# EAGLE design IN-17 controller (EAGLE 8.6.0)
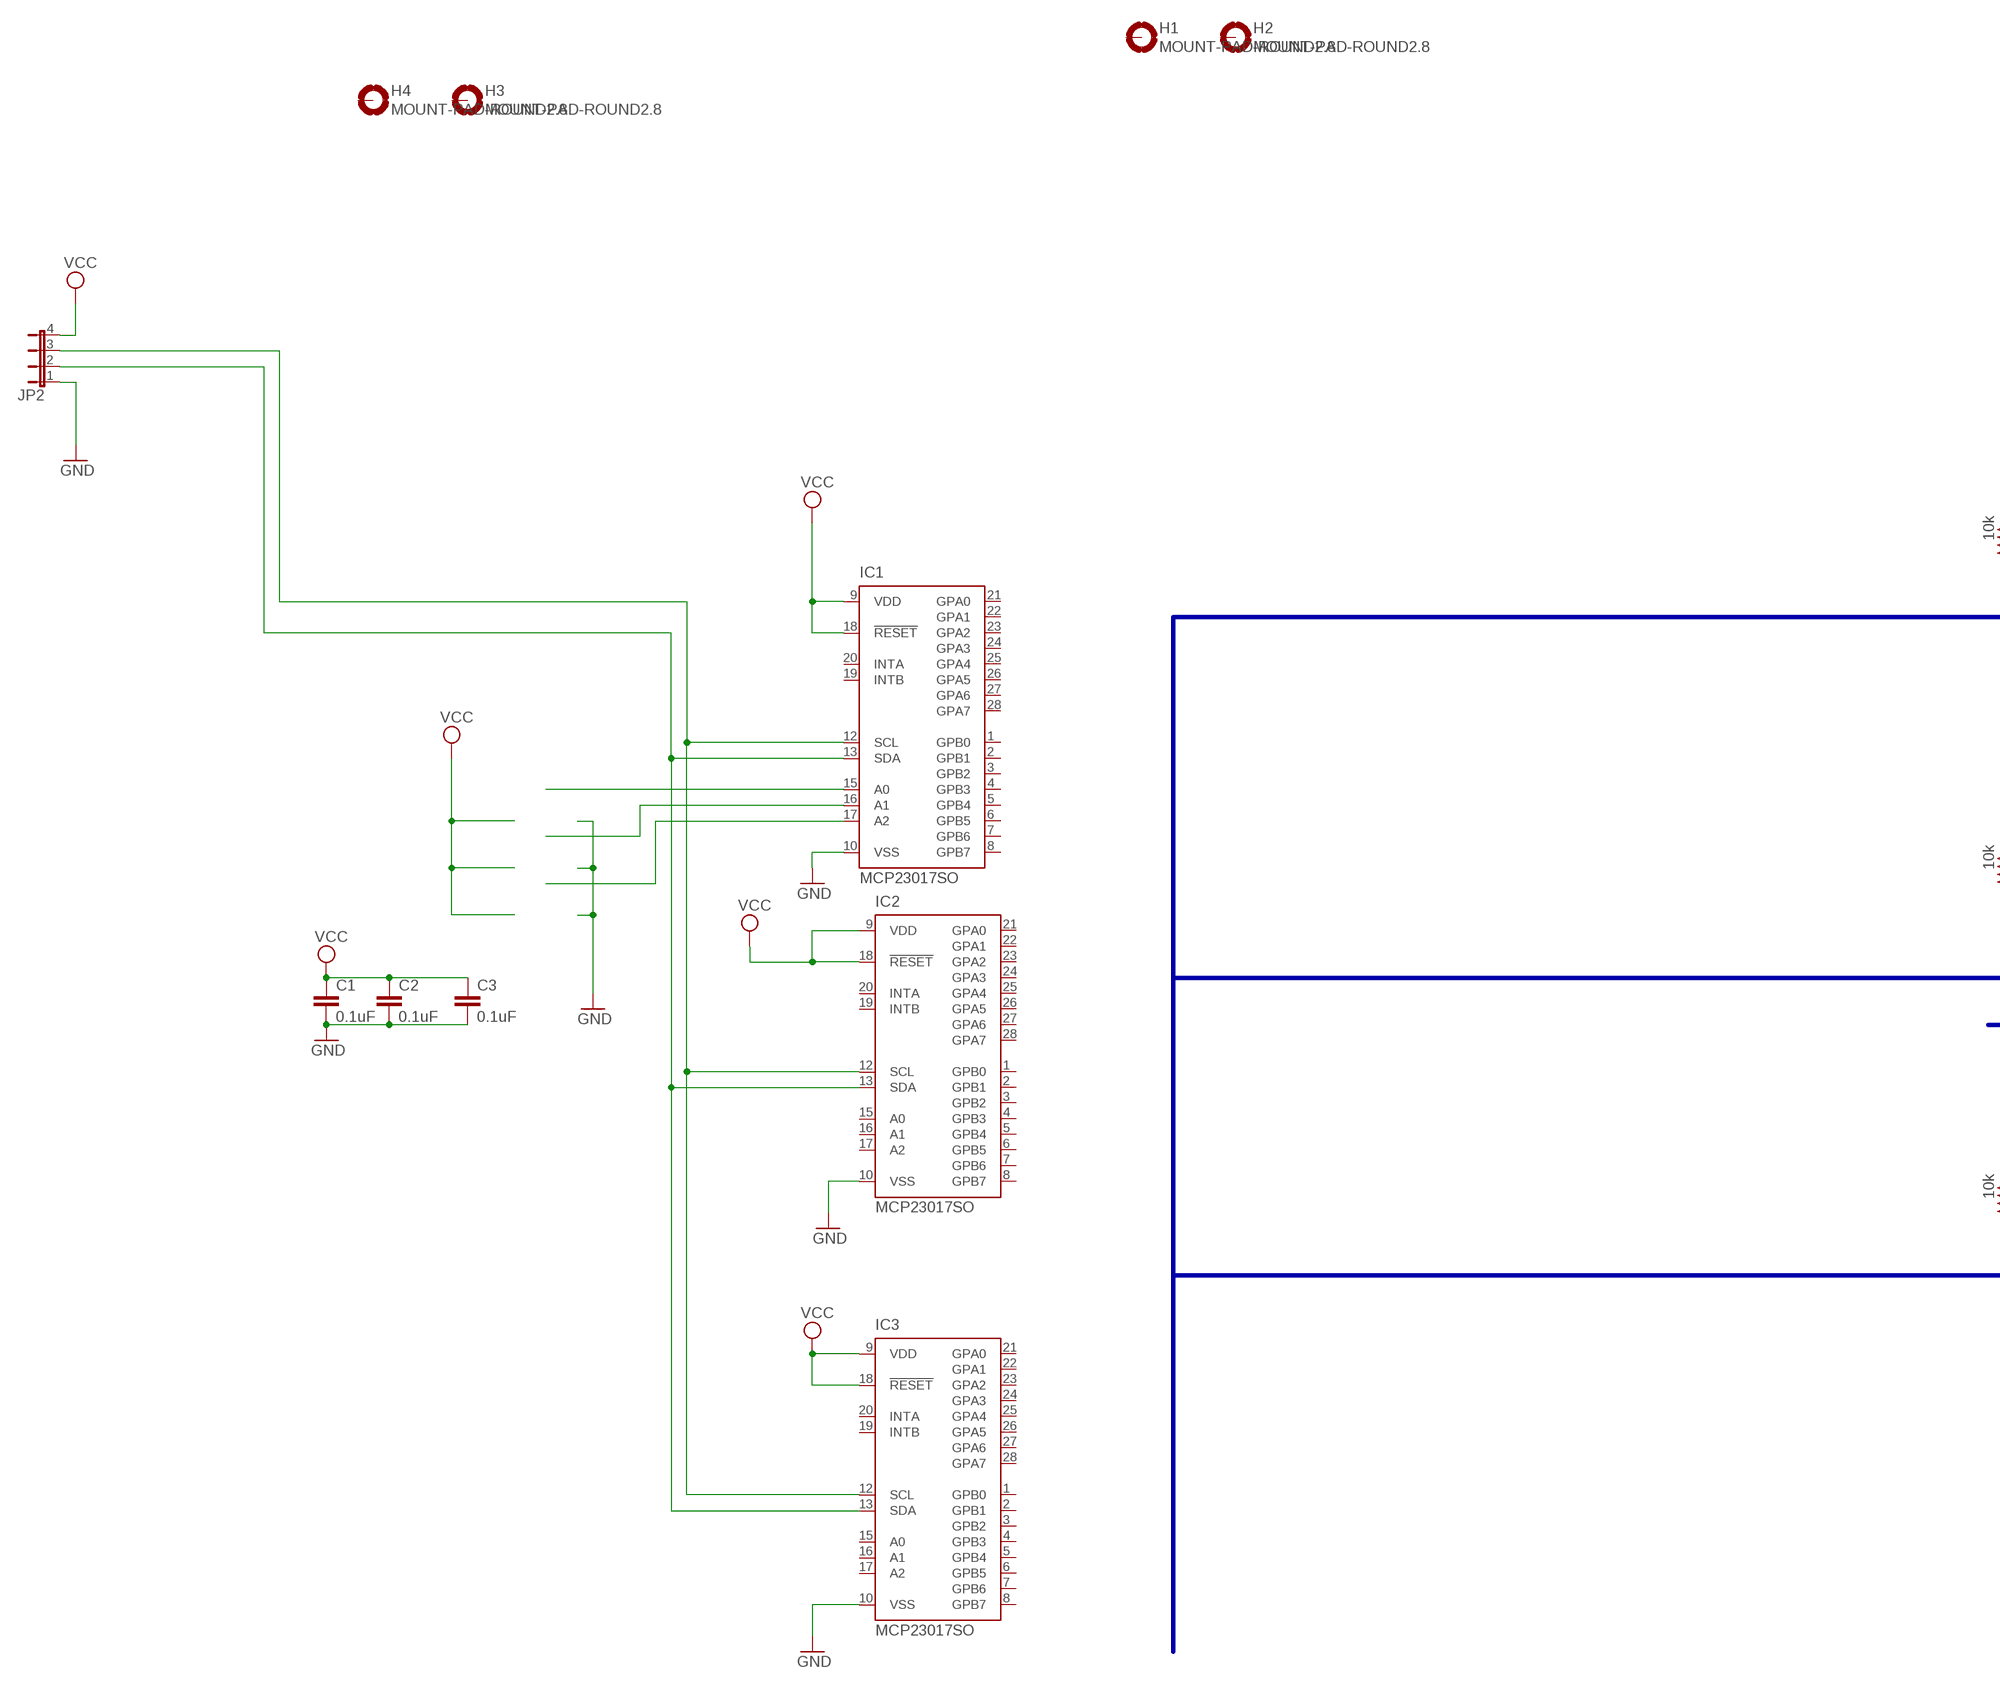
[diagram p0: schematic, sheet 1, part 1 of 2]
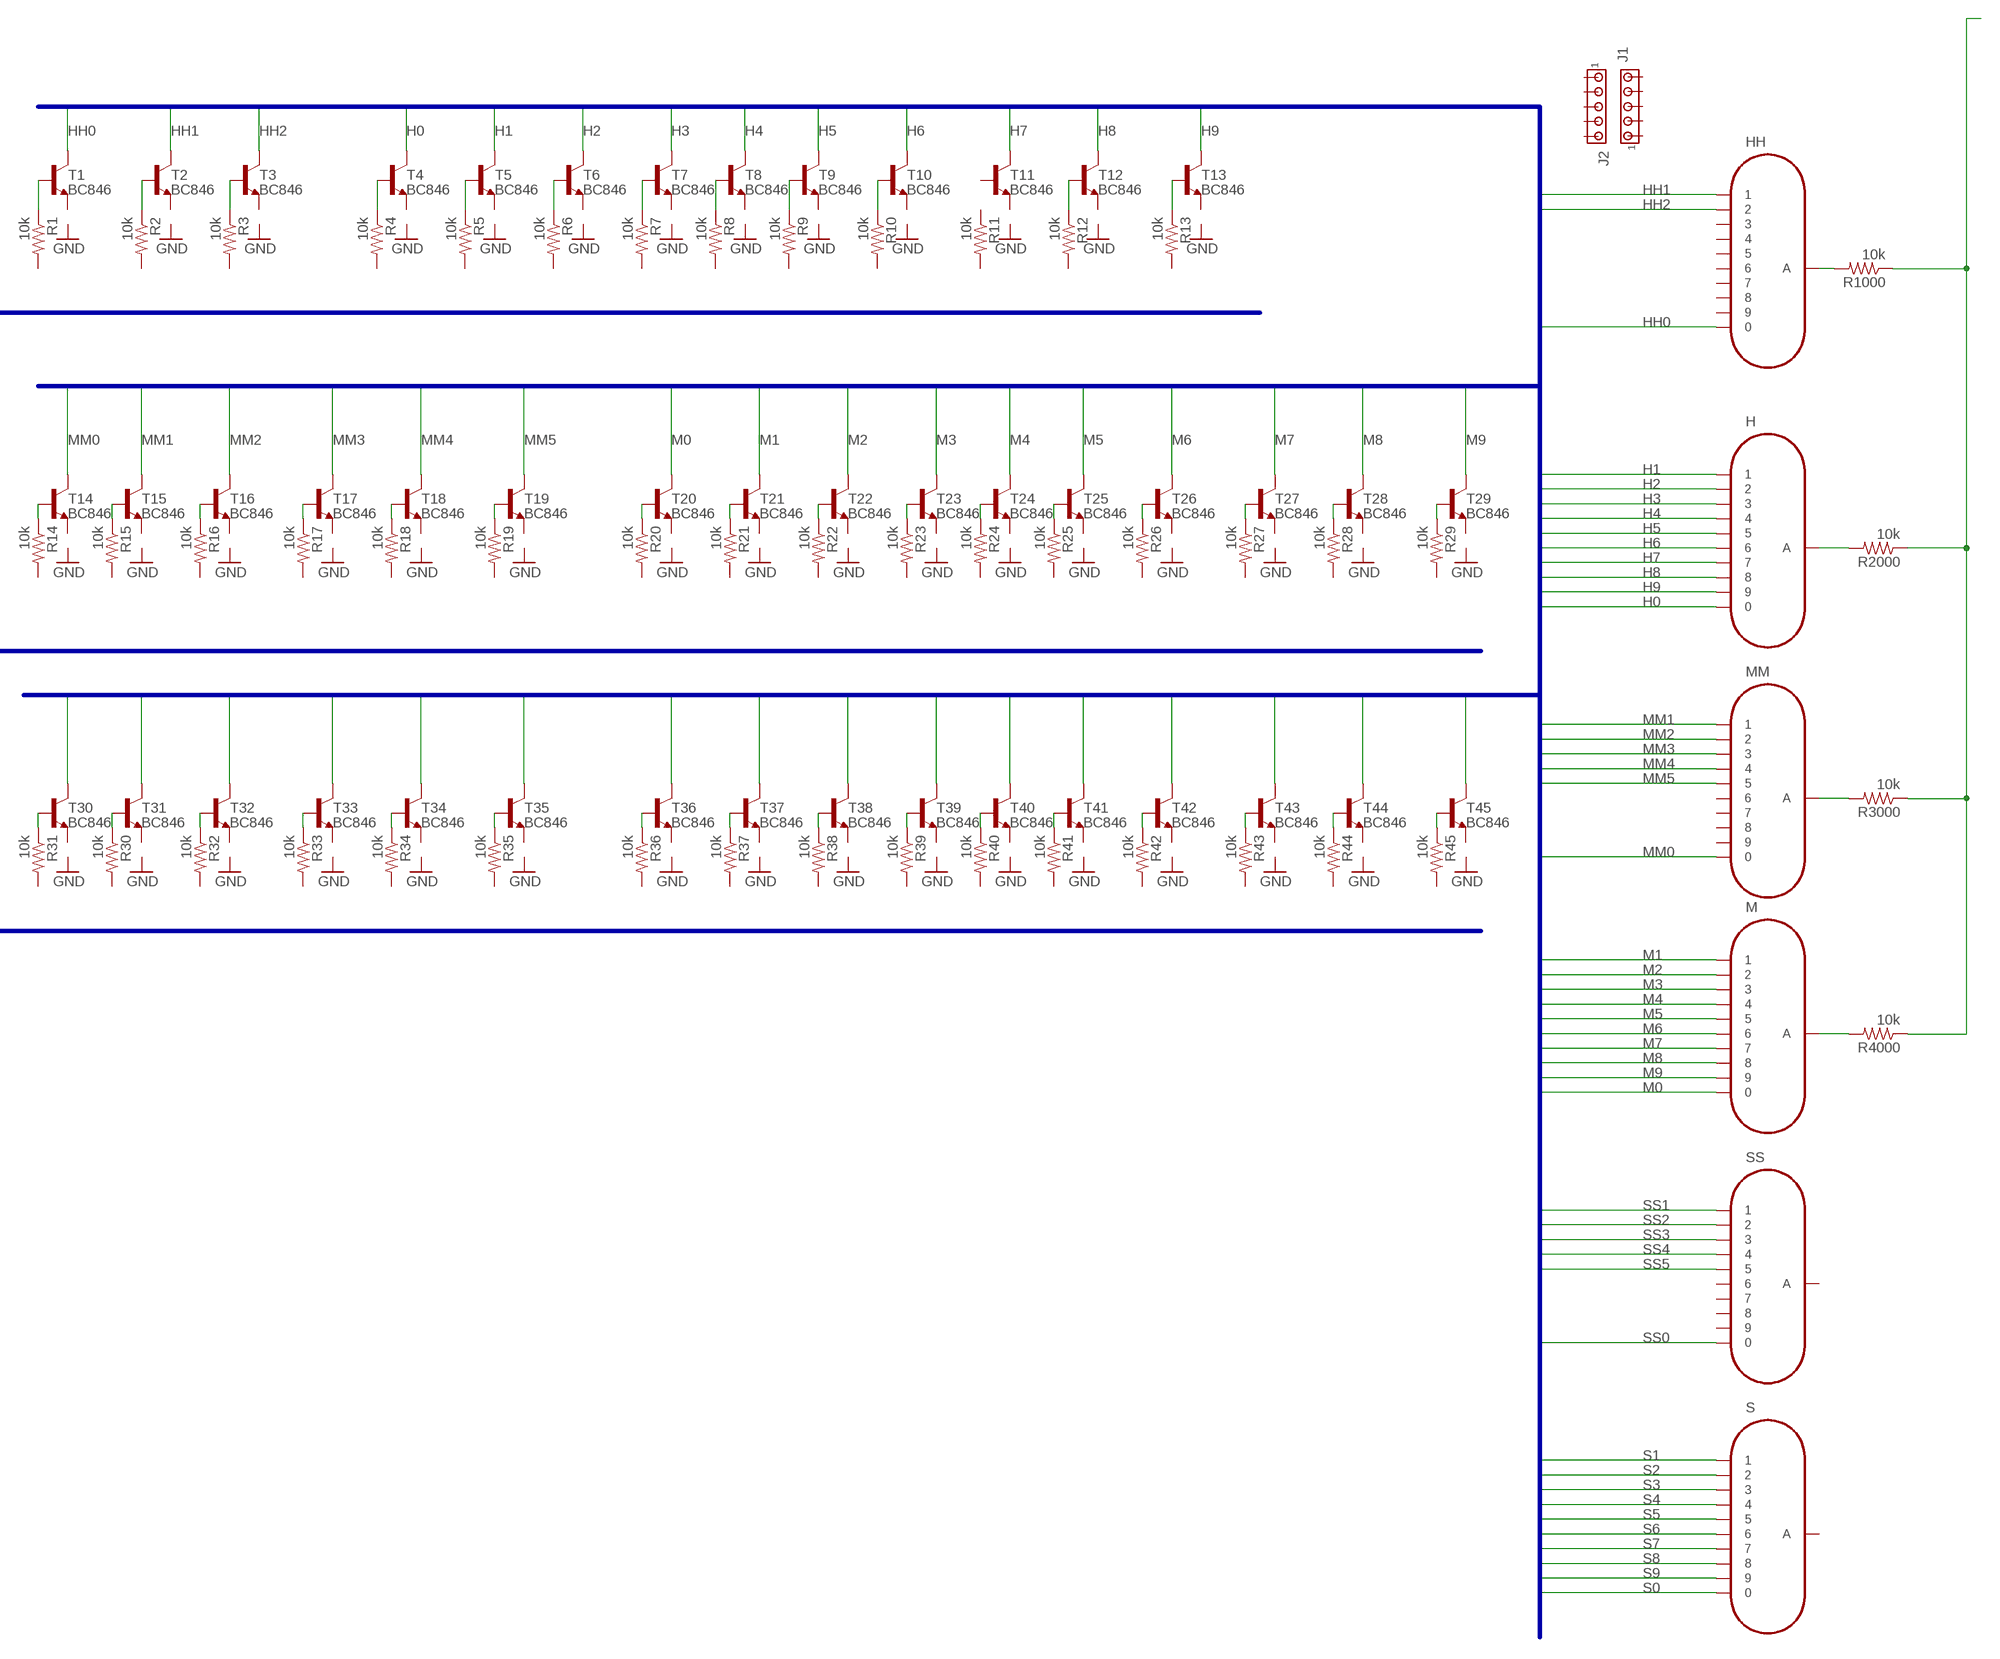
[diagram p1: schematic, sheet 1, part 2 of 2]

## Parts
C1  0.1uF  C-EUC1206  [C1206]
C2  0.1uF  C-EUC1206  [C1206]
C3  0.1uF  C-EUC1206  [C1206]
H  IN-17  [IN-17]
H1  MOUNT-PAD-ROUND2.8  [2,8-PAD]
H2  MOUNT-PAD-ROUND2.8  [2,8-PAD]
H3  MOUNT-PAD-ROUND2.8  [2,8-PAD]
H4  MOUNT-PAD-ROUND2.8  [2,8-PAD]
HH  IN-17  [IN-17]
IC1  MCP23017SO  [SO28W]
IC2  MCP23017SO  [SO28W]
IC3  MCP23017SO  [SO28W]
J1  MTA05-100  [10X05MTA]
J2  MTA05-100  [10X05MTA]
JP2  JP4E  [JP4]
M  IN-17  [IN-17]
MM  IN-17  [IN-17]
R1  10k  R-US_M0805  [M0805]
R2  10k  R-US_M0805  [M0805]
R3  10k  R-US_M0805  [M0805]
R4  10k  R-US_M0805  [M0805]
R5  10k  R-US_M0805  [M0805]
R6  10k  R-US_M0805  [M0805]
R7  10k  R-US_M0805  [M0805]
R8  10k  R-US_M0805  [M0805]
R9  10k  R-US_M0805  [M0805]
R10  10k  R-US_M0805  [M0805]
R11  10k  R-US_M0805  [M0805]
R12  10k  R-US_M0805  [M0805]
R13  10k  R-US_M0805  [M0805]
R14  10k  R-US_M0805  [M0805]
R15  10k  R-US_M0805  [M0805]
R16  10k  R-US_M0805  [M0805]
R17  10k  R-US_M0805  [M0805]
R18  10k  R-US_M0805  [M0805]
R19  10k  R-US_M0805  [M0805]
R20  10k  R-US_M0805  [M0805]
R21  10k  R-US_M0805  [M0805]
R22  10k  R-US_M0805  [M0805]
R23  10k  R-US_M0805  [M0805]
R24  10k  R-US_M0805  [M0805]
R25  10k  R-US_M0805  [M0805]
R26  10k  R-US_M0805  [M0805]
R27  10k  R-US_M0805  [M0805]
R28  10k  R-US_M0805  [M0805]
R29  10k  R-US_M0805  [M0805]
R30  10k  R-US_M0805  [M0805]
R31  10k  R-US_M0805  [M0805]
R32  10k  R-US_M0805  [M0805]
R33  10k  R-US_M0805  [M0805]
R34  10k  R-US_M0805  [M0805]
R35  10k  R-US_M0805  [M0805]
R36  10k  R-US_M0805  [M0805]
R37  10k  R-US_M0805  [M0805]
R38  10k  R-US_M0805  [M0805]
R39  10k  R-US_M0805  [M0805]
R40  10k  R-US_M0805  [M0805]
R41  10k  R-US_M0805  [M0805]
R42  10k  R-US_M0805  [M0805]
R43  10k  R-US_M0805  [M0805]
R44  10k  R-US_M0805  [M0805]
R45  10k  R-US_M0805  [M0805]
R1000  10k  R-US_M0805  [M0805]
R2000  10k  R-US_M0805  [M0805]
R3000  10k  R-US_M0805  [M0805]
R4000  10k  R-US_M0805  [M0805]
S  IN-17  [IN-17]
SS  IN-17  [IN-17]
T1  BC846  [SOT23]
T2  BC846  [SOT23]
T3  BC846  [SOT23]
T4  BC846  [SOT23]
T5  BC846  [SOT23]
T6  BC846  [SOT23]
T7  BC846  [SOT23]
T8  BC846  [SOT23]
T9  BC846  [SOT23]
T10  BC846  [SOT23]
T11  BC846  [SOT23]
T12  BC846  [SOT23]
T13  BC846  [SOT23]
T14  BC846  [SOT23]
T15  BC846  [SOT23]
T16  BC846  [SOT23]
T17  BC846  [SOT23]
T18  BC846  [SOT23]
T19  BC846  [SOT23]
T20  BC846  [SOT23]
T21  BC846  [SOT23]
T22  BC846  [SOT23]
T23  BC846  [SOT23]
T24  BC846  [SOT23]
T25  BC846  [SOT23]
T26  BC846  [SOT23]
T27  BC846  [SOT23]
T28  BC846  [SOT23]
T29  BC846  [SOT23]
T30  BC846  [SOT23]
T31  BC846  [SOT23]
T32  BC846  [SOT23]
T33  BC846  [SOT23]
T34  BC846  [SOT23]
T35  BC846  [SOT23]
T36  BC846  [SOT23]
T37  BC846  [SOT23]
T38  BC846  [SOT23]
T39  BC846  [SOT23]
T40  BC846  [SOT23]
T41  BC846  [SOT23]
T42  BC846  [SOT23]
T43  BC846  [SOT23]
T44  BC846  [SOT23]
T45  BC846  [SOT23]

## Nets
GND: C1.2 C2.2 C3.2 IC1.10(VSS) IC2.10(VSS) IC3.10(VSS) JP2.1
H0: H.0 T4.3(C)
H1: H.1 T5.3(C)
H2: H.2 T6.3(C)
H3: H.3 T7.3(C)
H4: H.4 T8.3(C)
H5: H.5 T9.3(C)
H6: H.6 T10.3(C)
H7: H.7 T11.3(C)
H8: H.8 T12.3(C)
H9: H.9 T13.3(C)
HH0: HH.0 T1.3(C)
HH1: HH.1 T2.3(C)
HH2: HH.2 T3.3(C)
M0: M.0 T20.3(C)
M1: M.1 T21.3(C)
M2: M.2 T22.3(C)
M3: M.3 T23.3(C)
M4: M.4 T24.3(C)
M5: M.5 T25.3(C)
M6: M.6 T26.3(C)
M7: M.7 T27.3(C)
M8: M.8 T28.3(C)
M9: M.9 T29.3(C)
MM0: MM.0 T14.3(C)
MM1: MM.1 T15.3(C)
MM2: MM.2 T16.3(C)
MM3: MM.3 T17.3(C)
MM4: MM.4 T18.3(C)
MM5: MM.5 T19.3(C)
N$1: IC1.15(A0)
N$2: R4.1 T4.1(B)
N$3: R14.1 T14.1(B)
N$4: R5.1 T5.1(B)
N$5: R6.1 T6.1(B)
N$6: R1.1 T1.1(B)
N$7: R2.1 T2.1(B)
N$8: R3.1 T3.1(B)
N$9: M.A R4000.2
N$10: R7.1 T7.1(B)
N$11: R8.1 T8.1(B)
N$12: R9.1 T9.1(B)
N$13: R10.1 T10.1(B)
N$14: H.A R2000.2
N$15: R12.1 T12.1(B)
N$16: R13.1 T13.1(B)
N$17: MM.A R3000.2
N$18: R15.1 T15.1(B)
N$19: R16.1 T16.1(B)
N$20: R17.1 T17.1(B)
N$21: R18.1 T18.1(B)
N$22: R19.1 T19.1(B)
N$23: R20.1 T20.1(B)
N$24: R21.1 T21.1(B)
N$25: R22.1 T22.1(B)
N$26: R23.1 T23.1(B)
N$28: R24.1 T24.1(B)
N$29: R25.1 T25.1(B)
N$30: R26.1 T26.1(B)
N$31: R27.1 T27.1(B)
N$32: R28.1 T28.1(B)
N$33: R29.1 T29.1(B)
N$35: R31.1 T30.1(B)
N$36: R30.1 T31.1(B)
N$37: R32.1 T32.1(B)
N$38: R1000.1 R2000.1 R3000.1 R4000.1
N$39: R33.1 T33.1(B)
N$40: IC1.16(A1)
N$41: R34.1 T34.1(B)
N$42: R35.1 T35.1(B)
N$43: IC1.17(A2)
N$44: R36.1 T36.1(B)
N$45: R37.1 T37.1(B)
N$46: R38.1 T38.1(B)
N$47: R39.1 T39.1(B)
N$48: R40.1 T40.1(B)
N$49: JP2.4 ; supply symbol labelled VCC
N$50: HH.A R1000.2
N$51: R41.1 T41.1(B)
N$52: R42.1 T42.1(B)
N$53: R44.1 T44.1(B)
N$54: R45.1 T45.1(B)
N$55: R43.1 T43.1(B)
N$88: IC1.13(SDA) IC2.13(SDA) IC3.13(SDA) JP2.2
N$89: IC1.12(SCL) IC2.12(SCL) IC3.12(SCL) JP2.3
S0: S.0 T36.3(C)
S1: S.1 T37.3(C)
S2: S.2 T38.3(C)
S3: S.3 T39.3(C)
S4: S.4 T40.3(C)
S5: S.5 T41.3(C)
S6: S.6 T42.3(C)
S7: S.7 T43.3(C)
S8: S.8 T44.3(C)
S9: S.9 T45.3(C)
SS0: SS.0 T30.3(C)
SS1: SS.1 T31.3(C)
SS2: SS.2 T32.3(C)
SS3: SS.3 T33.3(C)
SS4: SS.4 T34.3(C)
SS5: SS.5 T35.3(C)
VCC: C1.1 C2.1 C3.1 IC1.9(VDD) IC1.18(!RESET) IC2.9(VDD) IC2.18(!RESET) IC3.9(VDD) IC3.18(!RESET)
Unconnected: H1.B2,8(MOUNT) H2.B2,8(MOUNT) H3.B2,8(MOUNT) H4.B2,8(MOUNT) HH.3 HH.4 HH.5 HH.6 HH.7 HH.8 HH.9 IC1.1(GPB0) IC1.2(GPB1) IC1.3(GPB2) IC1.4(GPB3) IC1.5(GPB4) IC1.6(GPB5) IC1.7(GPB6) IC1.8(GPB7) IC1.19(INTB) IC1.20(INTA) IC1.21(GPA0) IC1.22(GPA1) IC1.23(GPA2) IC1.24(GPA3) IC1.25(GPA4) IC1.26(GPA5) IC1.27(GPA6) IC1.28(GPA7) IC2.1(GPB0) IC2.2(GPB1) IC2.3(GPB2) IC2.4(GPB3) IC2.5(GPB4) IC2.6(GPB5) IC2.7(GPB6) IC2.8(GPB7) IC2.15(A0) IC2.16(A1) IC2.17(A2) IC2.19(INTB) IC2.20(INTA) IC2.21(GPA0) IC2.22(GPA1) IC2.23(GPA2) IC2.24(GPA3) IC2.25(GPA4) IC2.26(GPA5) IC2.27(GPA6) IC2.28(GPA7) IC3.1(GPB0) IC3.2(GPB1) IC3.3(GPB2) IC3.4(GPB3) IC3.5(GPB4) IC3.6(GPB5) IC3.7(GPB6) IC3.8(GPB7) IC3.15(A0) IC3.16(A1) IC3.17(A2) IC3.19(INTB) IC3.20(INTA) IC3.21(GPA0) IC3.22(GPA1) IC3.23(GPA2) IC3.24(GPA3) IC3.25(GPA4) IC3.26(GPA5) IC3.27(GPA6) IC3.28(GPA7) J1.1 J1.2 J1.3 J1.4 J1.5 J2.1 J2.2 J2.3 J2.4 J2.5 MM.6 MM.7 MM.8 MM.9 R1.2 R2.2 R3.2 R4.2 R5.2 R6.2 R7.2 R8.2 R9.2 R10.2 R11.1 R11.2 R12.2 R13.2 R14.2 R15.2 R16.2 R17.2 R18.2 R19.2 R20.2 R21.2 R22.2 R23.2 R24.2 R25.2 R26.2 R27.2 R28.2 R29.2 R30.2 R31.2 R32.2 R33.2 R34.2 R35.2 R36.2 R37.2 R38.2 R39.2 R40.2 R41.2 R42.2 R43.2 R44.2 R45.2 S.A SS.6 SS.7 SS.8 SS.9 SS.A T1.2(E) T2.2(E) T3.2(E) T4.2(E) T5.2(E) T6.2(E) T7.2(E) T8.2(E) T9.2(E) T10.2(E) T11.1(B) T11.2(E) T12.2(E) T13.2(E) T14.2(E) T15.2(E) T16.2(E) T17.2(E) T18.2(E) T19.2(E) T20.2(E) T21.2(E) T22.2(E) T23.2(E) T24.2(E) T25.2(E) T26.2(E) T27.2(E) T28.2(E) T29.2(E) T30.2(E) T31.2(E) T32.2(E) T33.2(E) T34.2(E) T35.2(E) T36.2(E) T37.2(E) T38.2(E) T39.2(E) T40.2(E) T41.2(E) T42.2(E) T43.2(E) T44.2(E) T45.2(E)

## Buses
HH[0..2],H[0..9],MM[0..5],M[0..9],SS[0..5],S[0..9]
THH[0..3],TH[0..9],TMM[0..5],TM[0..9],TSS[0..5],TS[0..9]

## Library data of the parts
C1-C3 = rcl:C-EU: CAPACITOR, European symbol
H HH M MM S SS = russian-nixies:IN-17: IN-17: tiny numeric topview nixie tube
H1-H4 = holes:MOUNT-PAD-ROUND: MOUNTING PAD, round
IC1-IC3 = adafruit:MCP23017: http://ww1.microchip.com/downloads/en/DeviceDoc/21952a.pdf Source: http://ww1.microchip.com/downloads/en/DeviceDoc/21952a.pdf
J1 J2 = con-amp:MTA05-100: AMP connector
JP2 = jumper:JP4E: JUMPER
R1-R45 R1000 R2000 R3000 R4000 = adafruit:R-US_: RESISTOR, American symbol
T1-T45 = transistor:BC846: NPN TRANSISTOR

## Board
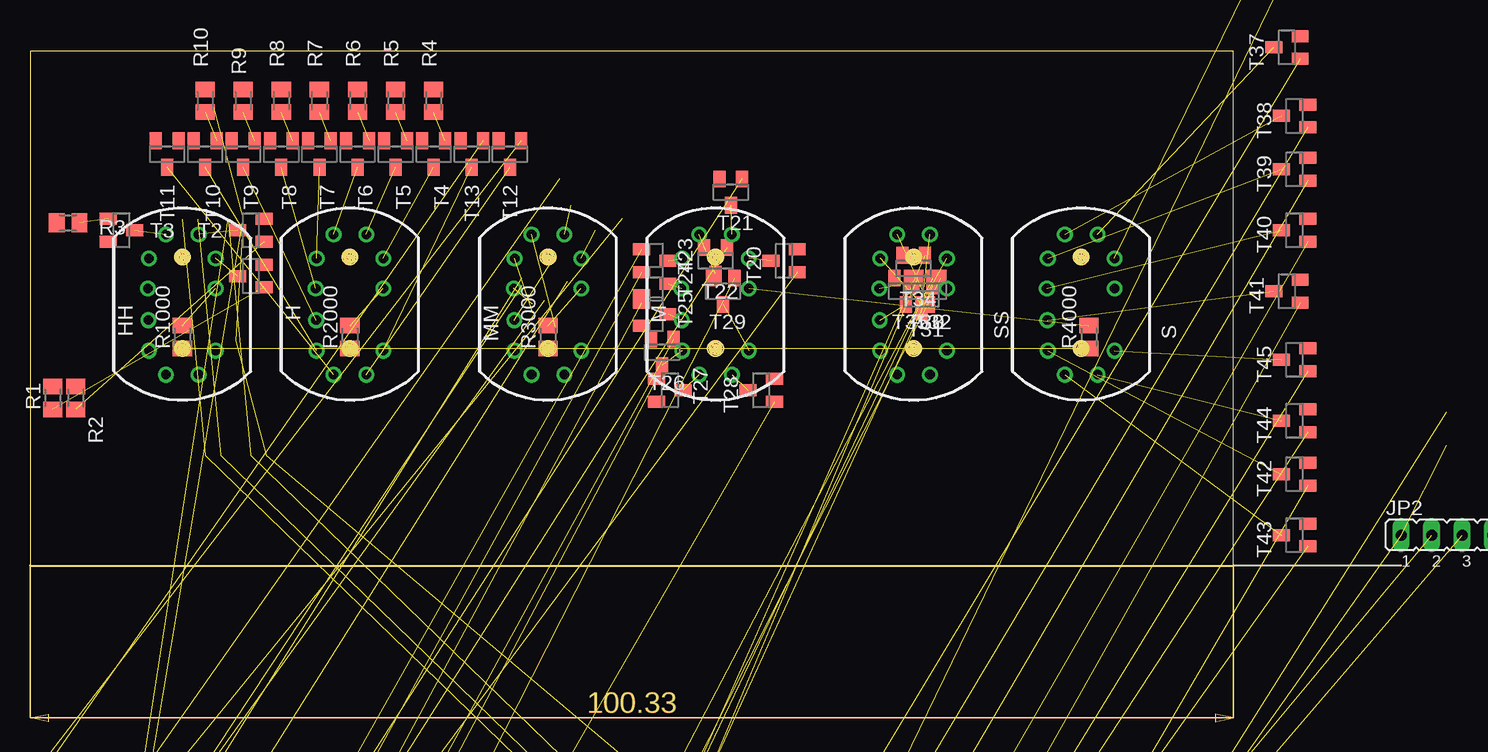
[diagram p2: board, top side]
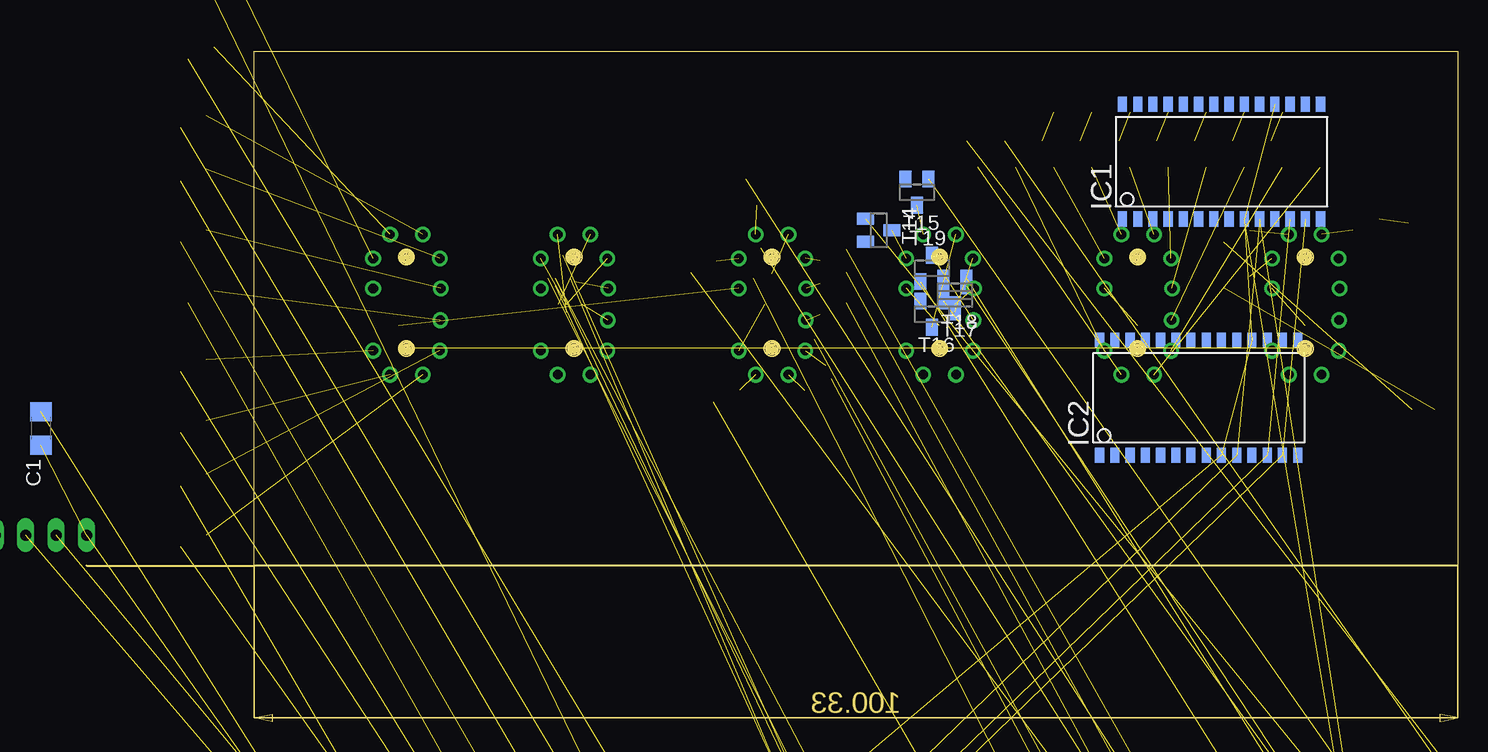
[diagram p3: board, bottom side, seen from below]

Size 114.3 x 55.85 mm. Coordinates in mm from the lower left corner, seen from the top.
Outline: 100.31,13 100.31,55.85 0,55.85 0,13 100.31,13
Outline: 114.3,13 100.31,13
Copper layers (1*16): Top 0.035mm / dielectric 1.5mm / Bottom 0.035mm
Design rules "default": minimum track width 10mil, minimum drill 24mil, track to track 8mil, track to pad 8mil, pad to pad 8mil, via to via 8mil, smd to smd 8mil, copper to edge 40mil, drill to drill 8mil, minimum pad ring 10mil, minimum via ring 8mil, stop-mask expansion 4mil, vias tented up to drill 0mil, thermal gap 10mil

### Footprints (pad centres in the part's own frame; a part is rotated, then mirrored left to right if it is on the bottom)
C1206 = smd 1.6 x 1.8: 1 -1.4,0; 2 1.4,0
IN-17 = drill 0.8: 0 2.777,4; 1 1.365,6; 2 -1.365,6; 3 -2.778,4; 4 -2.858,1.5; 5 -2.818,-1.143; 6 -2.778,-3.683; 7 -1.365,-5.683; 8 1.365,-5.683; 9 2.777,-3.683; A 2.777,1.5
2,8-PAD = drill 2.8 pad 5.334: B2,8 0,0
SO28W = smd 0.762 x 1.27: 1 -7.62,-4.78; 2 -6.35,-4.78; 3 -5.08,-4.78; 4 -3.81,-4.78; 5 -2.54,-4.78; 6 -1.27,-4.78; 7 0,-4.78; 8 1.27,-4.78; 9 2.54,-4.78; 10 3.81,-4.78; 11 5.08,-4.78; 12 6.35,-4.78; 13 7.62,-4.78; 14 8.89,-4.78; 15 8.89,4.78; 16 7.62,4.78; 17 6.35,4.78; 18 5.08,4.78; 19 3.81,4.78; 20 2.54,4.78; 21 1.27,4.78; 22 0,4.78; 23 -1.27,4.78; 24 -2.54,4.78; 25 -3.81,4.78; 26 -5.08,4.78; 27 -6.35,4.78; 28 -7.62,4.78
10X05MTA = drill 1.016 long: 1 5.08,0; 2 2.54,0; 3 0,0; 4 -2.54,0; 5 -5.08,0
JP4 = drill 0.914 long: 1 -3.81,0; 2 -1.27,0; 3 1.27,0; 4 3.81,0
M0805 = smd 1.3 x 1.6: 1 -0.95,0; 2 0.95,0
SOT23 = smd 1 x 1.4: 1 -0.95,-1.1; 2 0.95,-1.1; 3 0,1.1

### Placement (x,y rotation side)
C1  not placed on the board
C2  not placed on the board
C3  not placed on the board
H  26.67,34.59 0 top
H1  not placed on the board
H2  not placed on the board
H3  not placed on the board
H4  not placed on the board
HH  12.7,34.59 0 top
IC1  20.32,46.66 0 bottom
IC2  22.23,26.97 0 bottom
IC3  not placed on the board
J1  not placed on the board
J2  not placed on the board
JP2  118.11,15.54 0 top
M  57.15,34.59 0 top
MM  43.18,34.59 0 top
R1  1.91,26.97 90 top
R2  3.81,26.97 90 top
R3  3.17,41.58 180 top
R4  33.66,51.73 90 top
R5  30.48,51.73 90 top
R6  27.3,51.73 90 top
R7  24.13,51.73 90 top
R8  20.95,51.73 90 top
R9  17.78,51.73 90 top
R10  14.61,51.73 90 top
R11  not placed on the board
R12  not placed on the board
R13  not placed on the board
R14  not placed on the board
R15  not placed on the board
R16  not placed on the board
R17  not placed on the board
R18  not placed on the board
R19  not placed on the board
R20  not placed on the board
R21  not placed on the board
R22  not placed on the board
R23  not placed on the board
R24  not placed on the board
R25  not placed on the board
R26  not placed on the board
R27  not placed on the board
R28  not placed on the board
R29  not placed on the board
R30  not placed on the board
R31  not placed on the board
R32  not placed on the board
R33  not placed on the board
R34  not placed on the board
R35  not placed on the board
R36  not placed on the board
R37  not placed on the board
R38  not placed on the board
R39  not placed on the board
R40  not placed on the board
R41  not placed on the board
R42  not placed on the board
R43  not placed on the board
R44  not placed on the board
R45  not placed on the board
R1000  12.7,32.05 90 top
R2000  26.67,32.05 90 top
R3000  43.18,32.05 90 top
R4000  88.27,32.05 90 top
S  87.63,34.59 0 top
SS  73.66,34.59 0 top
T1  18.41,37.13 90 top
T2  18.41,40.94 90 top
T3  7.62,40.94 270 top
T4  33.66,47.29 180 top
T5  30.48,47.29 180 top
T6  27.3,47.29 180 top
T7  24.13,47.29 180 top
T8  20.95,47.29 180 top
T9  17.78,47.29 180 top
T10  14.61,47.29 180 top
T11  11.43,47.29 180 top
T12  40.01,47.29 180 top
T13  36.83,47.29 180 top
T14  48.26,40.94 270 bottom
T15  45.09,44.11 180 bottom
T16  43.81,33.95 180 bottom
T17  41.91,35.23 180 bottom
T18  41.91,35.86 180 bottom
T19  43.81,37.77 0 bottom
T20  62.87,38.4 90 top
T21  58.42,44.11 180 top
T22  57.15,38.4 180 top
T23  52.07,38.4 270 top
T24  52.07,36.5 270 top
T25  52.07,33.95 270 top
T26  52.7,30.78 180 top
T27  53.34,27.61 270 top
T28  60.96,27.61 90 top
T29  57.78,35.86 180 top
T30  74.3,35.86 180 top
T31  74.3,35.23 180 top
T32  74.93,35.86 180 top
T33  74.3,35.86 180 top
T34  73.66,37.77 180 top
T35  73.03,35.86 180 top
T36  not placed on the board
T37  104.78,56.18 90 top
T38  105.41,50.47 90 top
T39  105.41,46.02 90 top
T40  105.41,40.94 90 top
T41  104.78,35.86 90 top
T42  105.41,20.62 90 top
T43  105.41,15.54 90 top
T44  105.41,25.06 90 top
T45  105.41,30.14 90 top

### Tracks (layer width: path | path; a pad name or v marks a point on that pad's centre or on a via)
GND  (6 unrouted)
H0  (1 unrouted)
H1  (1 unrouted)
H2  (1 unrouted)
H3  (1 unrouted)
H4  (1 unrouted)
H5  (1 unrouted)
H6  (1 unrouted)
H7  (1 unrouted)
H8  (1 unrouted)
H9  (1 unrouted)
HH0  (1 unrouted)
  Top 0.203: HH.0 15.88,38.99
HH1  (1 unrouted)
HH2  (1 unrouted)
  Top 0.203: HH.2 10.98,40.94
M0  (1 unrouted)
M1  (1 unrouted)
M2  (1 unrouted)
M3  (1 unrouted)
M4  (1 unrouted)
M5  (1 unrouted)
M6  (1 unrouted)
M7  (1 unrouted)
M8  (1 unrouted)
M9  (1 unrouted)
MM0  (1 unrouted)
MM1  (1 unrouted)
MM2  (1 unrouted)
MM3  (1 unrouted)
MM4  (1 unrouted)
MM5  (1 unrouted)
N$2  (1 unrouted)
N$3  (1 unrouted)
N$4  (1 unrouted)
N$5  (1 unrouted)
N$6  (1 unrouted)
N$7  (1 unrouted)
N$8  (1 unrouted)
N$9  (1 unrouted)
N$10  (1 unrouted)
N$11  (1 unrouted)
N$12  (1 unrouted)
N$13  (1 unrouted)
N$14  (1 unrouted)
N$15  (1 unrouted)
N$16  (1 unrouted)
N$17  (1 unrouted)
N$18  (1 unrouted)
N$19  (1 unrouted)
N$20  (1 unrouted)
N$21  (1 unrouted)
N$22  (1 unrouted)
N$23  (1 unrouted)
N$24  (1 unrouted)
N$25  (1 unrouted)
N$26  (1 unrouted)
N$28  (1 unrouted)
N$29  (1 unrouted)
N$30  (1 unrouted)
N$31  (1 unrouted)
N$32  (1 unrouted)
N$33  (1 unrouted)
N$35  (1 unrouted)
N$36  (1 unrouted)
N$37  (1 unrouted)
N$38  (3 unrouted)
N$39  (1 unrouted)
N$41  (1 unrouted)
N$42  (1 unrouted)
N$44  (1 unrouted)
N$45  (1 unrouted)
N$46  (1 unrouted)
N$47  (1 unrouted)
N$48  (1 unrouted)
N$50  (1 unrouted)
N$51  (1 unrouted)
N$52  (1 unrouted)
N$53  (1 unrouted)
N$54  (1 unrouted)
N$55  (1 unrouted)
N$88  (3 unrouted)
N$89  (3 unrouted)
S0  (1 unrouted)
S1  (1 unrouted)
S2  (1 unrouted)
S3  (1 unrouted)
S4  (1 unrouted)
S5  (1 unrouted)
S6  (1 unrouted)
S7  (1 unrouted)
S8  (1 unrouted)
S9  (1 unrouted)
SS0  (1 unrouted)
SS1  (1 unrouted)
SS2  (1 unrouted)
SS3  (1 unrouted)
SS4  (1 unrouted)
SS5  (1 unrouted)
VCC  (8 unrouted)

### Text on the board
Bottom: SteamClock | SteamClock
